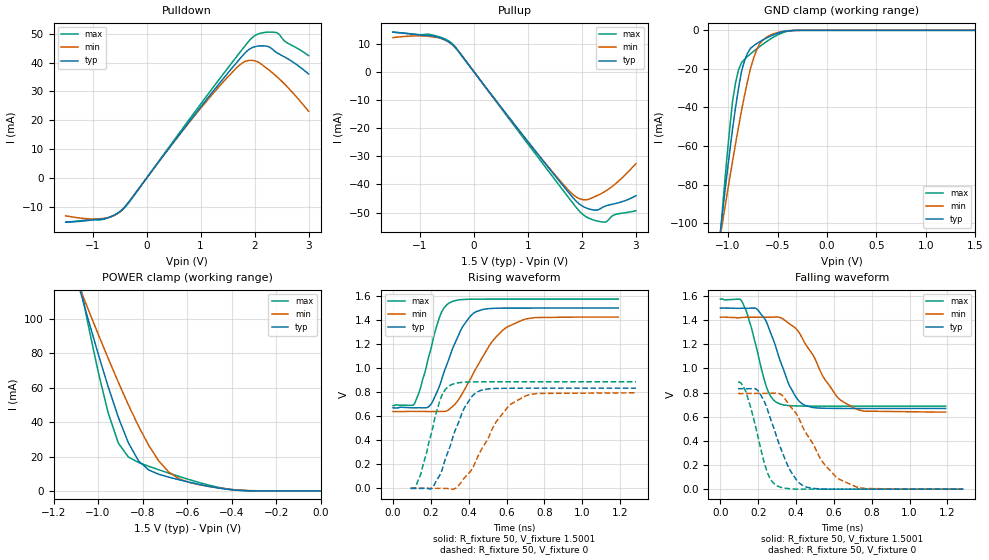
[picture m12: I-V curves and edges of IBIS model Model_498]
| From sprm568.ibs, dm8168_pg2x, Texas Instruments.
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| Model based on original model for BSHTLTCSCDDVGPBFZ
|   Sub model SLOWEST_10MA_5PER_N_1P5
[model]   Model_498
|[Description]  [1.5V-3-STATE-X-SLOWEST:10MA, IND, 5%]
|   Slowest slew rate (SR[1:0] = "11"), 0.80 * RExt = 1.250 * Iout
|   (I[2:0] = "101"), 10mA nominal with Rext = 50R, ,Industrial
|   temperature range (-40C to 125C, 25C nominal),5% power supply
|   tolerance
|[Input Load]
|[Output Drive] SLOWEST:10MA
|Voltage   1.5V
|Mode   3-STATE
Model_type   3-state
Polarity   Non-Inverting
Enable   Active-Low
Cref =  15.0000pF
Rref =  100.0000M
Vref =  0V
Vmeas =  0.75005
C_comp   1.5249p   1.4275p   1.6205p
[Model Spec]
[Temperature Range]   25   125   -40
[Voltage Range]   1.5   1.425   1.575
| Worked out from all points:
|   slope of the pulldown table from 0 to 0.225 V, typ, clamps not added: 39.9 ohm
|   slope of the pullup table from 0 to 0.225 V, typ, clamps not added: 39.8 ohm
|   GND clamp passes 1 mA (typ) near -0.47 V on its own axis
|   POWER clamp passes 1 mA (typ) near -0.42 V on its own axis
|   rising waveform, R_fixture 50, V_fixture 1.5001: 20-80 % time 123ps typ, 180ps min, 90ps max; typ from 0.669 V to 1.5 V
|   rising waveform, R_fixture 50, V_fixture 0: 20-80 % time 115ps typ, 170ps min, 87.8ps max; typ from 0 V to 0.834 V
|   falling waveform, R_fixture 50, V_fixture 1.5001: 20-80 % time 117ps typ, 176ps min, 87.7ps max; typ from 1.5 V to 0.669 V
|   falling waveform, R_fixture 50, V_fixture 0: 20-80 % time 118ps typ, 181ps min, 85.8ps max; typ from 0.833 V to 0 V
[POWER_clamp]
-1.5V     321.7mA    260.6mA    415.9mA
-1.076V   114.2mA    115.8mA    116.9mA
-1.061V   107.2mA    110.9mA    107.1mA
-954.6mV  60.59mA    77.06mA    45.35mA
-909.2mV  42.85mA    63.21mA    27.81mA
-863.7mV  27.9mA     49.99mA    19.69mA
-818.2mV  17.49mA    37.63mA    16.52mA
-772.8mV  12.19mA    26.53mA    14.33mA
-681.9mV  7.985mA    10.89mA    10.33mA
-590.9mV  5.094mA    4.955mA    6.6mA
-363.7mV  298.5uA    465.2uA    297.6uA
0V        1.518nA    24.08nA    367.8pA
[Pulldown]
-1.5V     -15.29mA   -13.07mA   -15.28mA
-772.8mV  -14.07mA   -13.9mA    -14.11mA
-590.9mV  -12.74mA   -12.86mA   -12.82mA
-409.1mV  -10.08mA   -10.11mA   -10.32mA
1.046V    25.68mA    25.17mA    26.75mA
1.591V    38.31mA    36.75mA    40.25mA
1.818V    43.24mA    40.36mA    45.69mA
1.955V    45.18mA    40.77mA    48.64mA
2.091V    45.77mA    39.91mA    50.06mA
2.273V    45.4mA     37.32mA    50.56mA
2.364V    44.07mA    35.93mA    50.51mA
3V        36.04mA    23.14mA    42.4mA
[Pullup]
-1.5V     14.1mA     12.18mA    14.13mA
-818.2mV  12.87mA    12.54mA    13.29mA
-590.9mV  11.83mA    11.72mA    12.11mA
-409.1mV  9.844mA    9.773mA    10.15mA
1.227V    -30.36mA   -30.27mA   -31.43mA
1.727V    -42.29mA   -41.55mA   -44.05mA
1.909V    -46.29mA   -44.65mA   -48.54mA
2.046V    -48.11mA   -45.48mA   -51.1mA
2.227V    -49.12mA   -44.44mA   -52.74mA
2.409V    -47.87mA   -42.71mA   -53.43mA
2.591V    -46.92mA   -40.26mA   -50.87mA
3V        -44.02mA   -32.61mA   -49.35mA
[GND_clamp]
-1.5V     -310.1mA   -250.5mA   -402.5mA
-1.076V   -103.6mA   -106.2mA   -105.2mA
-1.046V   -89.81mA   -96.36mA   -86.02mA
-954.6mV  -51.22mA   -67.87mA   -36.88mA
-924.3mV  -40.08mA   -58.86mA   -27.29mA
-863.7mV  -21.24mA   -41.56mA   -16.73mA
-833.4mV  -15.8mA    -33.75mA   -15.03mA
-772.8mV  -9.345mA   -19.75mA   -12.19mA
-712.2mV  -6.928mA   -10.35mA   -9.704mA
-621.3mV  -4.261mA   -3.896mA   -6.225mA
-409.1mV  -337.1uA   -289.1uA   -618.9uA
1.5V      1.518nA    257.2nA    299pA
[Ramp]
dV/dt_f   0.665552/0.1725485n   0.63044/0.26973069n   0.71/0.12908649n
dV/dt_r 0.67150528/0.17522791n 0.64148776/0.26571247n 0.71207976/0.1283244n
R_load = 50
[Rising Waveform]
R_fixture = 50
V_fixture = 1.5001
V_fixture_min = 1.425
V_fixture_max = 1.575
0s        669.3mV    639.1mV    688.4mV
114.5ps   669.8mV    640mV      707.8mV
202.8ps   704.7mV    639mV      1.176V
253.3ps   886.8mV    639.6mV    1.454V
310.6ps   1.146V     675.8mV    1.553V
423.8ps   1.455V     954.7mV    1.574V
521.2ps   1.497V     1.216V     1.575V
602.9ps   1.5V       1.342V     1.575V
744.2ps   1.5V       1.42V      1.575V
1.19ns    1.5V       1.425V     1.575V
[Rising Waveform]
R_fixture = 50
V_fixture = 0
V_fixture_min = 0
V_fixture_max = 0
93.15ps   0V         0V         0V
143.7ps   0V         0V         106.9mV
207.9ps   3.541mV    0V         490.3mV
255.5ps   137.2mV    0V         763.5mV
305.1ps   367mV      -6.193mV   859.6mV
374.2ps   660.2mV    80.61mV    883.1mV
435ps     791.7mV    217.6mV    886mV
548.5ps   831.5mV    561.2mV    886.7mV
699.6ps   833.4mV    768.4mV    886.8mV
1.284ns   833.5mV    794.6mV    886.9mV
[Falling Waveform]
R_fixture = 50
V_fixture = 1.5001
V_fixture_min = 1.425
V_fixture_max = 1.575
0s        1.499V     1.425V     1.575V
113.7ps   1.499V     1.422V     1.555V
163.2ps   1.5V       1.424V     1.34V
230.9ps   1.419V     1.424V     911.5mV
307.7ps   1.101V     1.425V     710.4mV
365.2ps   857.1mV    1.369V     691.8mV
432ps     707.5mV    1.253V     688.3mV
613.3ps   668.9mV    772.1mV    687.7mV
712.5ps   668.7mV    666.5mV    687.7mV
1.19ns    668.6mV    638.1mV    687.6mV
[Falling Waveform]
R_fixture = 50
V_fixture = 0
V_fixture_min = 0
V_fixture_max = 0
93.15ps   832.6mV    793.6mV    886mV
134.1ps   831.4mV    793.2mV    807.8mV
199ps     814mV      793.8mV    432.3mV
253.4ps   637.8mV    793.5mV    118.5mV
308ps     384mV      792.9mV    21.53mV
427.2ps   38.4mV     543.9mV    0V
536.7ps   2.016mV    233.2mV    0V
632.3ps   0V         78.89mV    0V
760.1ps   0V         5.955mV    0V
1.284ns   0V         0V         0V
